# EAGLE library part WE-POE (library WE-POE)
Transformer for Power-over-Ethernet WE-PoE - Flyback converter transducer particularly for PoE PDs - Insulation voltage 1,5 kVAC/1 min - Input voltages 36V till 57V -- Flyback converters -- Power-over-Ethernet PDs
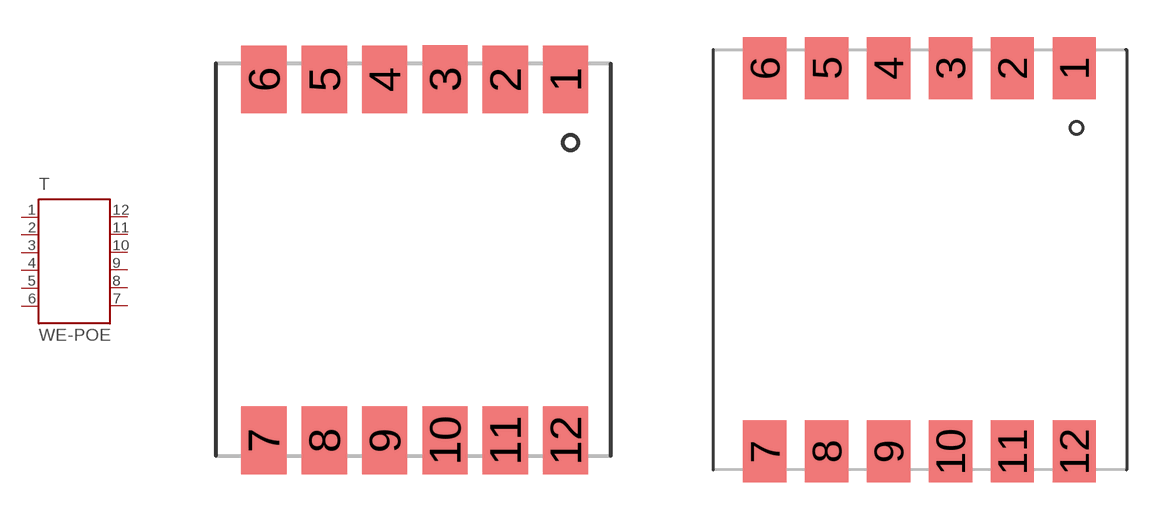
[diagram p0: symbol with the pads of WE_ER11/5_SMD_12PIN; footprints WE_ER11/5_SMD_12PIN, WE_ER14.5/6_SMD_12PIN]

Designator prefix T

## WE-POE_ER11/5, WE-POE-749119133_ER11/5 (MPN: 749119133; OC_FARNELL: 1848995; OC_NEWARK: 13T9803; PACKAGE: ER/11/5; SUPPLIER: Wuerth Elektronik), WE-POE-749119150_ER11/5 (MPN: 749119150; OC_FARNELL: 1848996; OC_NEWARK: 13T9804; PACKAGE: ER/11/5; SUPPLIER: Wuerth Elektronik)  [WE_ER11/5_SMD_12PIN]
1  1  pas
2  2  pas
3  3  pas
4  4  pas
5  5  pas
6  6  pas
7  7  pas
8  8  pas
9  9  pas
10  10  pas
11  11  pas
12  12  pas

## WE-POE_ER14.5/6, WE-POE-749119218_ER14.5/6 (MPN: 749119218; OC_FARNELL: 1848997; OC_NEWARK: 13T9805; PACKAGE: ER14.5/6; SUPPLIER: Wuerth Elektronik), WE-POE-749119233_ER14.5/6 (MPN: 749119233; OC_FARNELL: 1848998; OC_NEWARK: 13T9806; PACKAGE: ER14.5/6; SUPPLIER: Wuerth Elektronik), WE-POE-749119250_ER14.5/6 (MPN: 749119250; OC_FARNELL: 1849000; OC_NEWARK: 13T9807; PACKAGE: ER14.5/6; SUPPLIER: Wuerth Elektronik), WE-POE-7491192912_ER14.5/6 (MPN: 7491192912; OC_FARNELL: 1849002; OC_NEWARK: 13T9808; PACKAGE: ER14.5/6; SUPPLIER: Wuerth Elektronik)  [WE_ER14.5/6_SMD_12PIN]
Pads as for WE_ER11/5_SMD_12PIN

## WE-POE_EFD15, WE-POE-749119318_EFD15 (MPN: 749119318; OC_FARNELL: 1849003; OC_NEWARK: 13T9809; PACKAGE: EFD15; SUPPLIER: Wuerth Elektronik), WE-POE-749119333_EFD15 (MPN: 749119333; OC_FARNELL: 1849004; OC_NEWARK: 13T9810; PACKAGE: EFD15; SUPPLIER: Wuerth Elektronik), WE-POE-749119350_EFD15 (MPN: 749119350; OC_FARNELL: 1849005; OC_NEWARK: 13T9811; PACKAGE: EFD15; SUPPLIER: Wuerth Elektronik), WE-POE-7491193912_EFD15 (MPN: 7491193912; OC_FARNELL: 1849006; OC_NEWARK: 13T9812; PACKAGE: EFD15; SUPPLIER: Wuerth Elektronik)  [WE_EFD15_SMD_12PIN]
Pads as for WE_ER11/5_SMD_12PIN

## Footprint WE_ER11/5_SMD_12PIN (pad centres in mm)
Transformer, ER11/5 SMD 12Pin
smd 1.5 x 2.25: 1 4.92,5.9; 2 2.92,5.9; 3 0.92,5.91; 4 -1.08,5.9; 5 -3.08,5.9; 6 -5.08,5.9; 7 -5.08,-6.07; 8 -3.08,-6.07; 9 -1.08,-6.07; 10 0.92,-6.07; 11 2.92,-6.07; 12 4.92,-6.07

## Footprint WE_ER14.5/6_SMD_12PIN (pad centres in mm)
Transformer, ER14.5/6 SMD 12Pin
smd 1.75 x 2.5: 1 6.26,7.75; 2 3.76,7.75; 3 1.26,7.75; 4 -1.24,7.75; 5 -3.74,7.75; 6 -6.24,7.75; 7 -6.24,-7.75; 8 -3.74,-7.75; 9 -1.24,-7.75; 10 1.26,-7.75; 11 3.76,-7.75; 12 6.26,-7.75

## Footprint WE_EFD15_SMD_12PIN (pad centres in mm)
Transformer, EFD15 SMD 12 Pin
smd 2.62 x 1.17: 1 -9.895,6.225; 2 -9.895,3.735; 3 -9.895,1.245; 4 -9.895,-1.245; 5 -9.895,-3.735; 6 -9.895,-6.225; 7 9.895,-6.225; 8 9.895,-3.735; 9 9.895,-1.245; 10 9.895,1.245; 11 9.895,3.735; 12 9.895,6.225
